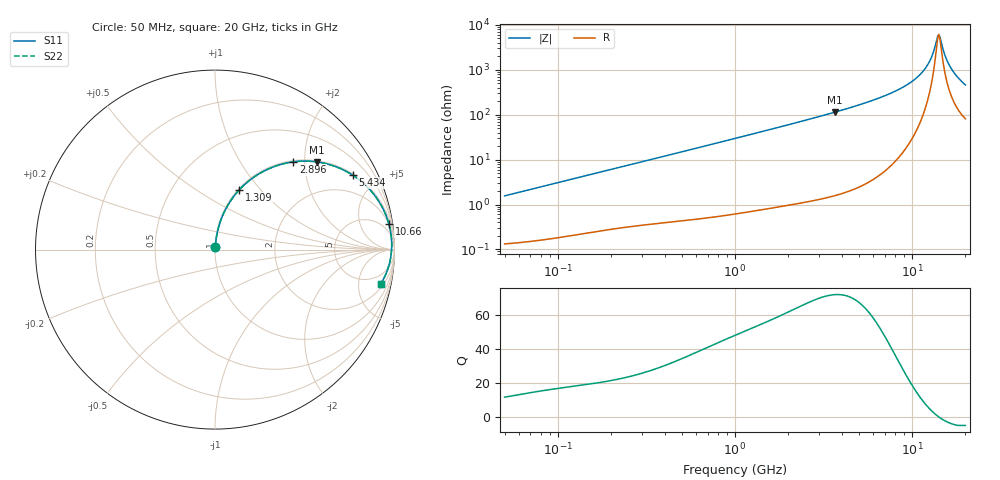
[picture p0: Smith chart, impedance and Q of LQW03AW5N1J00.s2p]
!Murata Part Number: LQW03AW5N1J00
!These Parameters are Measured in Series Mode Connection
!  o--[Z]--o
!Port1  Port2
!  o-------o
!Freq. Start=50[MHz] Stop=20[GHz], 401[Steps]
# Hz S RI R 50
!Freq.(Hz) S11(Real) S11(Imag) S21(Real) S21(Imag) S12(Real) S12(Imag) S22(Real) S22(Imag)
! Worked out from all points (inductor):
!   401 points, 50 MHz to 20 GHz, reference 50 ohm
!   read as one part in series: L = 4.93 nH near 51.52 MHz
!   highest Q = 72.3 at 3.681 GHz (marker M1), where L = 4.95 nH
!   self-resonance near 13.96 GHz
!   S11 on the Smith chart (normalised r, x): 50 MHz: 1.00, +0.03; 1.309 GHz: 1.01, +0.78; 2.896 GHz: 1.03, +1.76; 5.434 GHz: 1.06, +3.66; 10.66 GHz: 2, +13; 20 GHz: 2.62, -9.05
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5e7  0.00156 0.0155  0.9984 -0.0155  0.9984 -0.0155  0.00156 0.0155
1.364002e8  0.00393 0.0414  0.9961 -0.0414  0.9961 -0.0414  0.00393 0.0414
3.721004e8  0.0158 0.1088  0.9842 -0.1088  0.9842 -0.1088  0.0158 0.1088
1e9  0.0853 0.2691  0.9147 -0.2691  0.9147 -0.2691  0.0853 0.2691
1.309461e9  0.1355 0.333  0.8645 -0.333  0.8645 -0.333  0.1355 0.333
2.728004e9  0.4064 0.4839  0.5936 -0.4839  0.5936 -0.4839  0.4064 0.4839
2.896447e9  0.4371 0.4889  0.5629 -0.4889  0.5629 -0.4889  0.4371 0.4889
3.680849e9  0.5661 0.4887  0.4339 -0.4887  0.4339 -0.4887  0.5661 0.4887
5.433528e9  0.7666 0.4153  0.2334 -0.4153  0.2334 -0.4153  0.7666 0.4153
7.442007e9  0.889 0.3026  0.111 -0.3026  0.111 -0.3026  0.889 0.3026
9.178299e9  0.9437 0.2116  0.0563 -0.2116  0.0563 -0.2116  0.9437 0.2116
1.066139e10  0.969 0.1417  0.031 -0.1417  0.031 -0.1417  0.969 0.1417
1.166392e10  0.9786 0.0982  0.0214 -0.0982  0.0214 -0.0982  0.9786 0.0982
1.238412e10  0.9826 0.0685  0.0174 -0.0685  0.0174 -0.0685  0.9826 0.0685
1.295331e10  0.9842 0.0459  0.0158 -0.0459  0.0158 -0.0459  0.9842 0.0459
1.375312e10  0.9846 0.0152  0.0154 -0.0152  0.0154 -0.0152  0.9846 0.0152
1.417136e10  0.9839 -0.000304  0.0161 0.000304  0.0161 0.000304  0.9839 -0.000304
1.460232e10  0.9827 -0.016  0.0173 0.016  0.0173 0.016  0.9827 -0.016
1.550395e10  0.9783 -0.0479  0.0217 0.0479  0.0217 0.0479  0.9783 -0.0479
1.646126e10  0.9712 -0.0804  0.0288 0.0804  0.0288 0.0804  0.9712 -0.0804
1.800918e10  0.9545 -0.1304  0.0455 0.1304  0.0455 0.1304  0.9545 -0.1304
2e10  0.9237 -0.1905  0.0763 0.1905  0.0763 0.1905  0.9237 -0.1905
